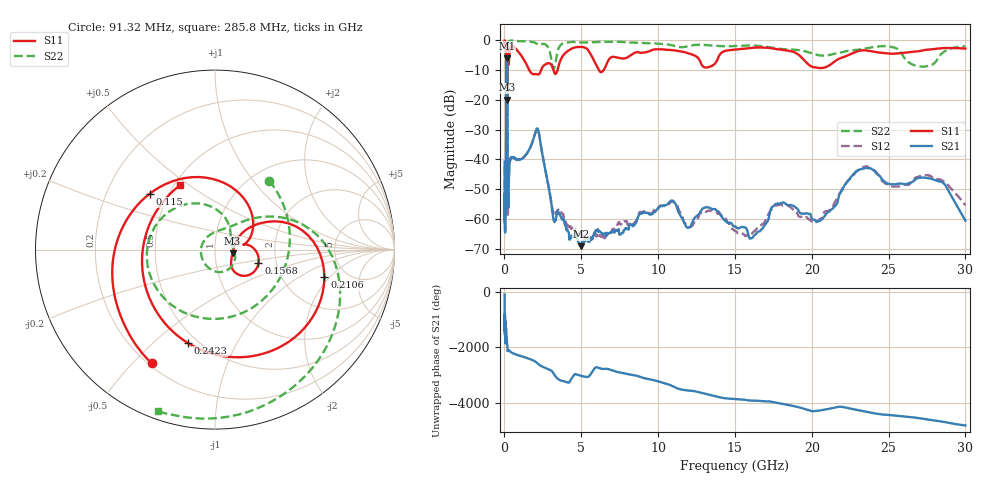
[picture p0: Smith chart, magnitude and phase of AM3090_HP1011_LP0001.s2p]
! Date/Time: Thu, Feb 28, 2019 2:05 PM
! Network Analyzer: Agilent Technologies E8364B Rev: A.07.50.67
! Sweep from 0.010 to 30.000 GHz, 1601 Points, Sweep Type: LOG
! Power Supply: 5.023 V, 0.002 A
# Hz S DB R 50
!freq MagS11 AngS11 MagS21 AngS21 MagS12 AngS12 MagS22 AngS22
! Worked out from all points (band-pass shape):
!   1601 points, 10 MHz to 30 GHz, reference 50 ohm
!   highest |S21| = -6.18 dB at 151.4 MHz (marker M1); lowest = -69.1 dB at 4.977 GHz (marker M2)
!   |S21| within 3 dB of the highest: 128.8 MHz to 181.5 MHz (52.68 MHz wide, 33.9 % of centre)
!   lowest |S11| = -20.0 dB at 183.1 MHz (marker M3), VSWR 1.22, Z = 60.8 - j2.47 ohm
!   |S11| at or under -10 dB: 1.609 GHz to 2.387 GHz (777.6 MHz wide, 38.9 % of centre); 3.186 GHz to 3.459 GHz (272.9 MHz wide, 8.21 % of centre); 6.142 GHz to 6.465 GHz (322.6 MHz wide, 5.12 % of centre)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
!   |S22| runs from -22.2 to -0.1 dB; largest |S21 - S12| = 0.016
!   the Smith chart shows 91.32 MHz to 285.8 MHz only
!   S11 on the Smith chart (normalised r, x): 91.32 MHz: 0.21, -0.57; 115 MHz: 0.39, +0.32; 156.8 MHz: 1.61, -0.26; 210.6 MHz: 3.43, -1.75; 242.3 MHz: 0.44, -0.65; 285.8 MHz: 0.54, +0.46
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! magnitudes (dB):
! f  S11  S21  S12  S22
! 10 MHz  -0.2  -40.7  -42.4  -0.6
! 38.04 MHz  -0.4  -61.3  -59.6  -1.3
! 49.84 MHz  -0.7  -49.4  -51.5  -1.3
! 91.32 MHz  -2.8  -56.7  -55.1  -6.2
! 115 MHz  -6.4  -22.8  -22.8  -8.2
! 144.7 MHz  -14.4  -6.3  -6.2  -19.6
! 151.4 MHz  -12.6  -6.2  -6.1  -17.9
! 156.8 MHz  -11.9  -6.2  -6.2  -17.6
! 183.1 MHz  -20.0  -9.8  -9.7  -17.3
! 210.6 MHz  -4.0  -49.7  -49.9  -2.4
! 242.3 MHz  -5.3  -54.6  -55.5  -0.7
! 285.8 MHz  -7.8  -46.9  -47.1  -0.4
! 550.5 MHz  -2.1  -39.5  -39.3  -0.2
! 2.084 GHz  -11.4  -30.0  -29.9  -1.2
! 3.22 GHz  -10.6  -60.5  -58.8  -9.6
! 4.977 GHz  -2.3  -69.1  -64.6  -0.8
! 7.926 GHz  -6.0  -63.4  -60.6  -0.8
! 10.76 GHz  -3.3  -54.1  -54.6  -1.6
! 15.81 GHz  -2.8  -63.9  -65.3  -1.8
! 20.82 GHz  -9.2  -59.1  -57.6  -5.2
! 23.48 GHz  -3.5  -42.9  -42.4  -2.9
! 30 GHz  -2.8  -60.5  -55.3  -2.1
